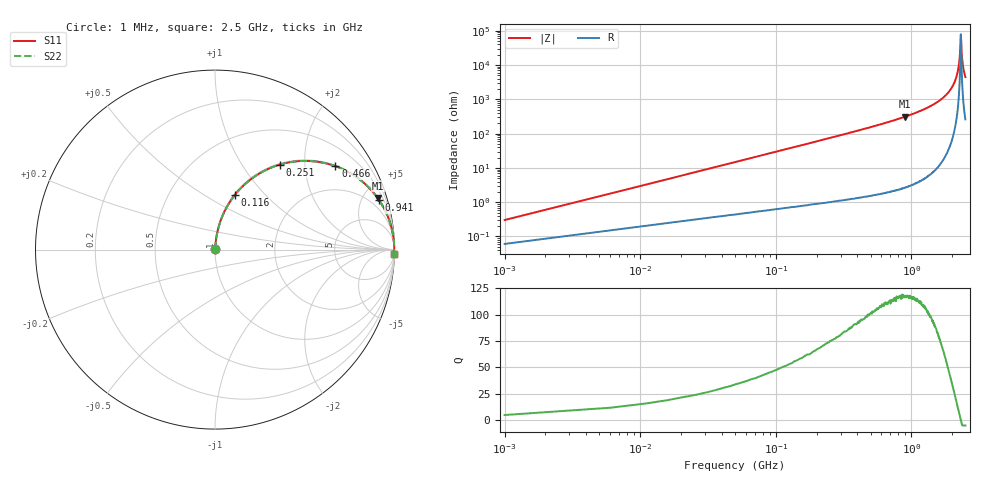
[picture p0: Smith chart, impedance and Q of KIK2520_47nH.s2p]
!version-2
!date-01.2022
!Series
# MHz S RI R 50
!Freq ReS11 ImS11 ReS21 ImS21 ReS12 ImS12 ReS22 ImS22
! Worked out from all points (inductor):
!   501 points, 1 MHz to 2.5 GHz, reference 50 ohm
!   read as one part in series: L = 47 nH near 11 MHz
!   highest Q = 117 at 901 MHz (marker M1), where L = 55.4 nH
!   self-resonance near 2.315 GHz
!   S11 on the Smith chart (normalised r, x): 1 MHz: 1.00, +0.01; 116 MHz: 1.01, +0.69; 251 MHz: 1.02, +1.50; 466 MHz: 1.03, +2.87; 941 MHz: 1.06, +6.66; 2.5 GHz: 6, -89
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1  0.000629 0.00295  0.9994 -0.00295  0.9994 -0.00295  0.000629 0.00295
16  0.00469 0.0469  0.9953 -0.0469  0.9953 -0.0469  0.00469 0.0469
31  0.0117 0.0902  0.9883 -0.0902  0.9883 -0.0902  0.0117 0.0902
66  0.0411 0.1861  0.9589 -0.1861  0.9589 -0.1861  0.0411 0.1861
116  0.1102 0.3035  0.8898 -0.3035  0.8898 -0.3035  0.1102 0.3035
251  0.3618 0.4739  0.6382 -0.4739  0.6382 -0.4739  0.3618 0.4739
421  0.6219 0.4796  0.3781 -0.4796  0.3781 -0.4796  0.6219 0.4796
466  0.6713 0.4647  0.3287 -0.4647  0.3287 -0.4647  0.6713 0.4647
836  0.8875 0.3117  0.1125 -0.3117  0.1125 -0.3117  0.8875 0.3117
901  0.9057 0.2881  0.0944 -0.2881  0.0944 -0.2881  0.9057 0.2881
941  0.9152 0.2743  0.0848 -0.2743  0.0848 -0.2743  0.9152 0.2743
1255  0.9634 0.183  0.0365 -0.183  0.0365 -0.183  0.9634 0.183
1670  0.9893 0.096  0.0107 -0.096  0.0107 -0.096  0.9893 0.096
1915  0.9956 0.0555  0.00437 -0.0555  0.00437 -0.0555  0.9956 0.0555
2085  0.9978 0.0305  0.0022 -0.0305  0.0022 -0.0305  0.9978 0.0305
2175  0.9984 0.0182  0.0016 -0.0182  0.0016 -0.0182  0.9984 0.0182
2240  0.9986 0.00961  0.00136 -0.00961  0.00136 -0.00961  0.9986 0.00961
2275  0.9987 0.00509  0.0013 -0.00509  0.0013 -0.00509  0.9987 0.00509
2315  0.9987 1.01e-05  0.00128 -1.01e-05  0.00128 -1.01e-05  0.9987 1.01e-05
2355  0.9987 -0.00498  0.00131 0.00498  0.00131 0.00498  0.9987 -0.00498
2385  0.9986 -0.00868  0.00136 0.00868  0.00136 0.00868  0.9986 -0.00868
2500  0.9982 -0.0223  0.00181 0.0223  0.00181 0.0223  0.9982 -0.0223
